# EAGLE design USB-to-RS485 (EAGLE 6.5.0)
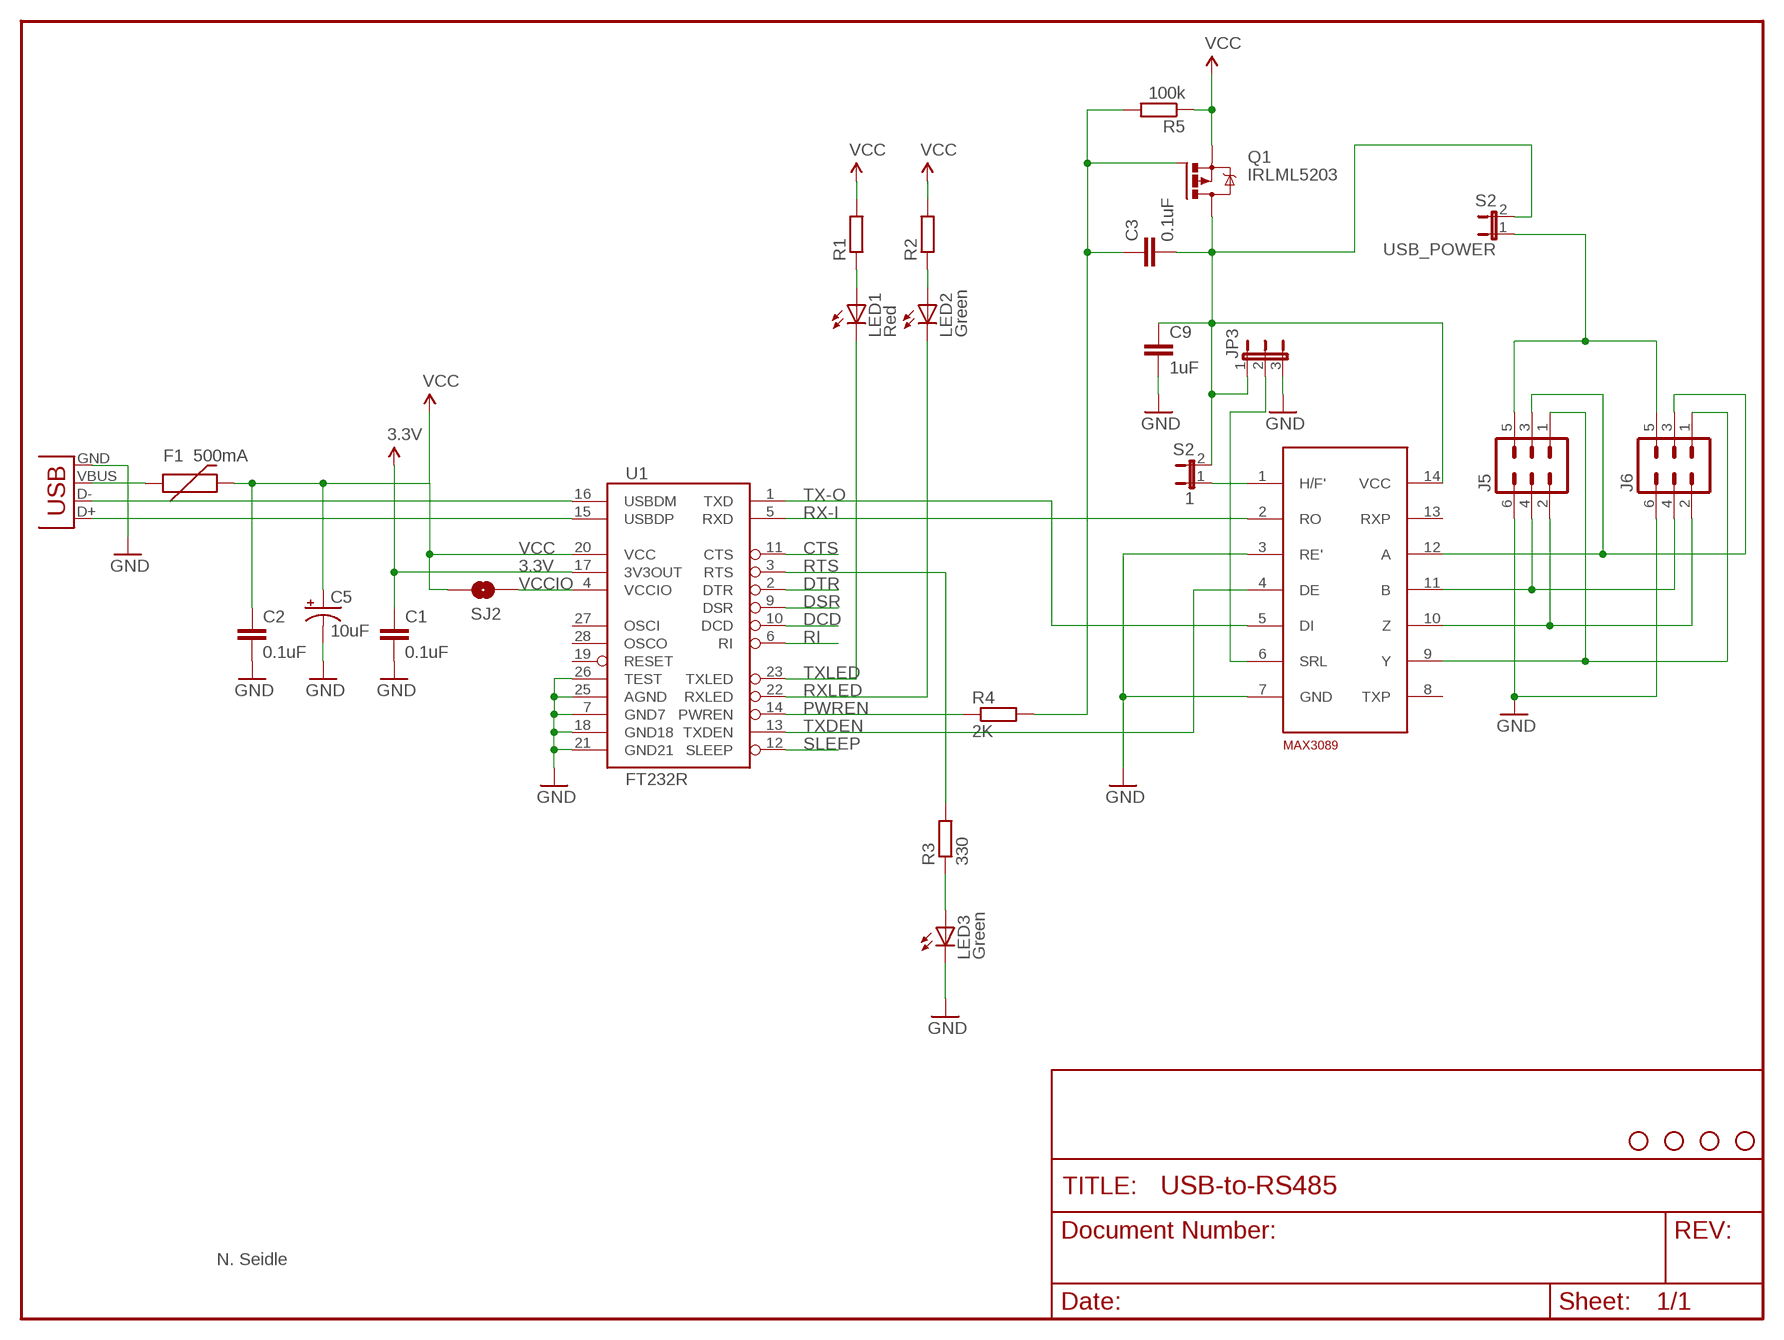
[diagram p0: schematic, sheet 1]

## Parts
1  S2  JP1E  [JP1]
C1  0.1uF  RCL_C-EUC0603  [RCL_C0603]
C2  0.1uF  RCL_C-EUC0603  [RCL_C0603]
C3  0.1uF  RCL_C-EUC0603  [RCL_C0603]
C5  10uF  CAP_POL1206  [EIA3216]
C9  1uF  RCL_C-EUC0603  [RCL_C0603]
F1  500mA  PTCSMD  [PTC-1206]
J5  ML6  [ML6]
J6  ML6  [ML6]
JP1  STAND-OFF  [STAND-OFF]
JP3  JP2E  [JP2]
JP6  STAND-OFF  [STAND-OFF]
JP7  STAND-OFF  [STAND-OFF]
JP8  STAND-OFF  [STAND-OFF]
LED1  Red  LED0603  [LED-0603]
LED2  Green  LED0603  [LED-0603]
LED3  Green  LED0603  [LED-0603]
Q1  IRLML5203  [MICRO3]
R1  RCL_R-EU_R0603  [RCL_R0603]
R2  RCL_R-EU_R0603  [RCL_R0603]
R3  330  RCL_R-EU_R0603  [RCL_R0603]
R4  2K  RCL_R-EU_R0603  [RCL_R0603]
R5  100k  RCL_R-EU_R0603  [RCL_R0603]
SJ2  SOLDERJUMPERNC2  [SJ_2S-NOTRACE]
U1  FT232R  FT232RLSSOP  [SSOP28DB]
U$4  MAX3089  [SO14]
USB_POWER  S2  JP1E  [JP1]
X2  USBSMD  [USB-MINIB]

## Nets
3.3V [power]: C1.1 U1.17(3V3OUT)
CTS: U1.11(CTS)
DCD: U1.10(DCD)
DSR: U1.9(DSR)
DTR: U1.2(DTR)
GND [power]: C1.2 C2.2 C5.C(-) C9.2 J5.6 J6.6 JP3.3 LED3.C U1.7(GND7) U1.18(GND18) U1.21(GND21) U1.25(AGND) U1.26(TEST) U$4.3(RE') U$4.7(GND) X2.GND
J5 [power]: J5.1 J6.1 U$4.9(Y)
N$1: LED1.A R1.1
N$2: LED2.A R2.1
N$3: F1.1 X2.VBUS
N$4: LED3.A R3.1
N$5 [power]: 1.2 C3.2 C9.1 JP3.1 Q1.3(D) U$4.14(VCC) USB_POWER.2
N$6 [supply]: J5.5 J6.5 USB_POWER.1
N$7: C3.1 Q1.1(G) R4.2 R5.2
N$9: JP3.2 U$4.6(SRL)
N$38 [supply]: 1.1 U$4.1(H/F')
N$41 [power]: J5.2 J6.2 U$4.10(Z)
N$48 [power]: J5.3 J6.3 U$4.12(A)
N$49 [power]: J5.4 J6.4 U$4.11(B)
PWREN: R4.1 U1.14(PWREN)
RI: U1.6(RI)
RTS: R3.2 U1.3(RTS)
RX-I: U1.5(RXD) U$4.2(RO)
RXLED: LED2.C U1.22(RXLED)
SLEEP: U1.12(SLEEP)
TX-O: U1.1(TXD) U$4.5(DI)
TXDEN: U1.13(TXDEN) U$4.4(DE)
TXLED: LED1.C U1.23(TXLED)
USB_D+: U1.15(USBDP) X2.D+
USB_D-: U1.16(USBDM) X2.D-
VCC [power]: C2.1 C5.A(+) F1.2 Q1.2(S) R1.2 R2.2 R5.1 SJ2.2 U1.20(VCC)
VCCIO: SJ2.1 U1.4(VCCIO)
Unconnected: U1.19(RESET) U1.27(OSCI) U1.28(OSCO) U$4.8(TXP) U$4.13(RXP)

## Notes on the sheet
- N. Seidle

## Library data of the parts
1 USB_POWER = jumper:JP1E: JUMPER
C1-C3 C9 = mc_rip2_1:RCL_C-EU: CAPACITOR, European symbol
C5 = SparkFun:CAP_POL: Capacitor Polarized
F1 = SparkFun:PTC: Resettable Fuse PTC
J5 J6 = con-harting-ml:ML6: HARTING
JP1 JP6-JP8 = SparkFun:STAND-OFF: Stand Off
JP3 = jumper:JP2E: JUMPER
LED1-LED3 = SparkFun:LED: LEDs
Q1 = transistor-power:IRLML5203: HEXFET P-Channel Power MOSFET
R1-R5 = mc_rip2_1:RCL_R-EU_: RESISTOR, European symbol
SJ2 = SparkFun:SOLDERJUMPER: Solder Jumper
U1 = SparkFun:FT232RL: USB UART FT232RL 4th Generation USB UART (USB <-> Serial) Controller. Spark Fun Electronics SKU : COM-00650
U$4 = maxim:MAX3089: RS485 driver
X2 = SparkFun:USB: USB Connectors USB-B-PTH is fully proven SKU : PRT-00139 USB-miniB is fully proven SKU : PRT-00587 USB-A-PCB is untested. USB-A-H is throughly reviewed, but untested. Spark Fun Electronics SKU : PRT-00437 USB-B-SMT is throughly reviewed, but untested. Needs silkscreen touching up. USB-A-S has not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

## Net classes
0 default: width 0.203 mm
1 power: width 0.254 mm
2 supply: width 0.5 mm, clearance 0.2 mm

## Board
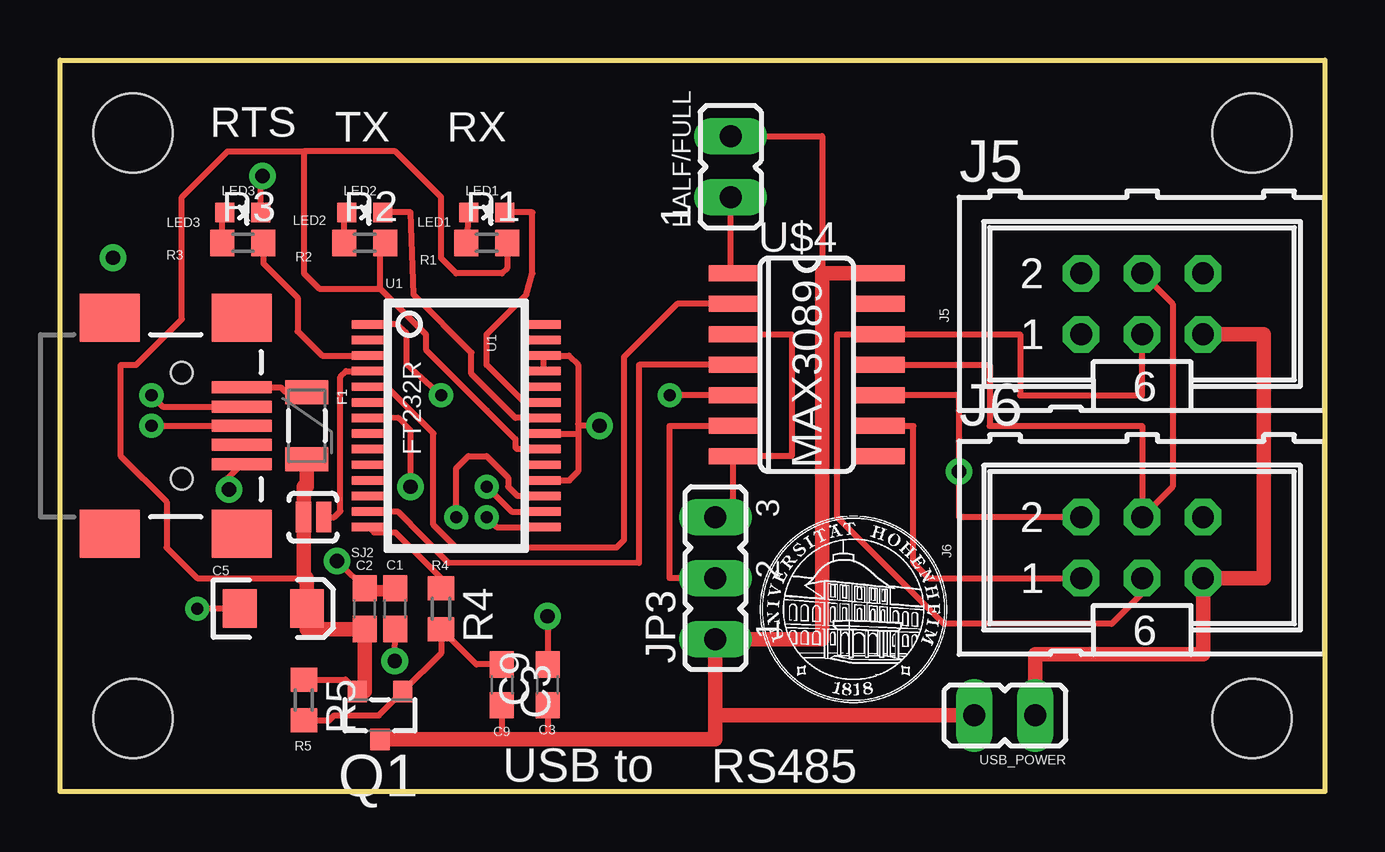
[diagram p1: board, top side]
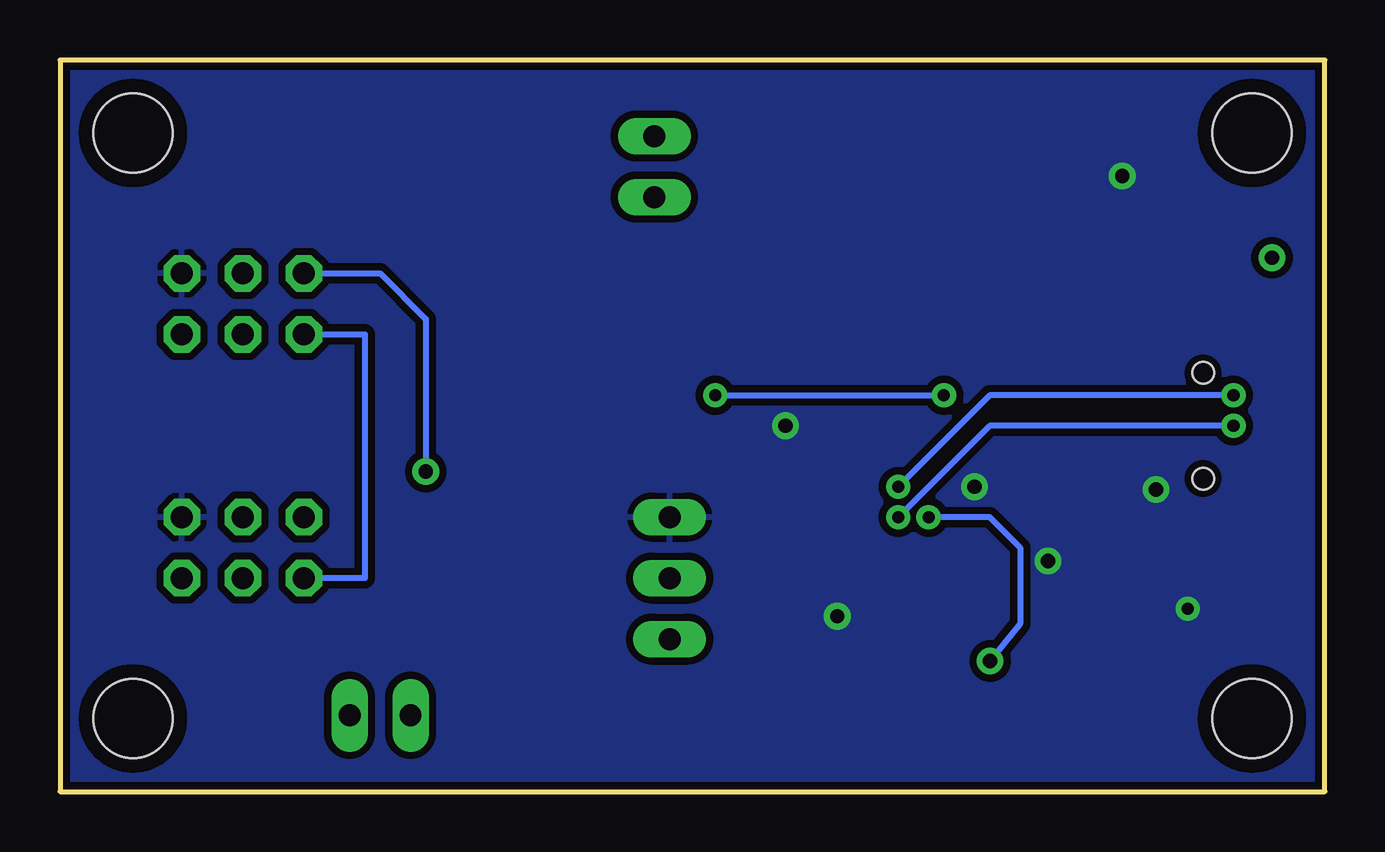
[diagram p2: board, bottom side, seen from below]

Size 52.7 x 30.48 mm. Coordinates in mm from the lower left corner, seen from the top.
Outline: 52.7,0 0,0 0,30.48 52.7,30.48 52.7,0
Copper layers (1*16): Top 0.035mm / dielectric 1.5mm / Bottom 0.035mm
Design rules "SparkFun": minimum track width 8mil, minimum drill 20mil, track to track 8mil, track to pad 8mil, pad to pad 8mil, via to via 8mil, smd to smd 8mil, copper to edge 8mil, drill to drill 8mil, minimum pad ring 12mil, minimum via ring 10mil, stop-mask expansion 4mil, vias tented up to drill 20mil, thermal gap 10mil

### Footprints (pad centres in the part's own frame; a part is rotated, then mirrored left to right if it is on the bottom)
JP1 = drill 0.914 long: 1 0,-1.27; 2 0,1.27
RCL_C0603 = smd 1.1 x 1: 1 -0.85,0; 2 0.85,0
EIA3216 = smd 1.4 x 1.6: A 1.4,0; C -1.4,0
PTC-1206 = smd 1 x 1.8: 1 -1.4,0; 2 1.4,0
ML6 = drill 0.914 octagon: 1 -2.54,-1.27; 2 -2.54,1.27; 3 0,-1.27; 4 0,1.27; 5 2.54,-1.27; 6 2.54,1.27
STAND-OFF = hole 3.302: 0,0
JP2 = drill 0.914 long: 1 -2.54,0; 2 0,0; 3 2.54,0
LED-0603 = smd 0.8 x 0.8: A 0,-0.75; C 0,0.75
MICRO3 = smd 0.8 x 0.9: 1 -0.95,-1; 2 0.95,-1; 3 0,1
RCL_R0603 = smd 1 x 1.1: 1 -0.85,0; 2 0.85,0
SJ_2S-NOTRACE = smd 0.635 x 1.27: 1 -0.45,0; 2 0.4,0
SSOP28DB = smd 0.348 x 1.397: 1 -4.225,-3.656; 2 -3.575,-3.656; 3 -2.925,-3.656; 4 -2.275,-3.656; 5 -1.625,-3.656; 6 -0.975,-3.656; 7 -0.325,-3.656; 8 0.325,-3.656; 9 0.975,-3.656; 10 1.625,-3.656; 11 2.275,-3.656; 12 2.925,-3.656; 13 3.575,-3.656; 14 4.225,-3.656; 15 4.225,3.656; 16 3.575,3.656; 17 2.925,3.656; 18 2.275,3.656; 19 1.625,3.656; 20 0.975,3.656; 21 0.325,3.656; 22 -0.325,3.656; 23 -0.975,3.656; 24 -1.625,3.656; 25 -2.275,3.656; 26 -2.925,3.656; 27 -3.575,3.656; 28 -4.225,3.656
SO14 = smd 0.66 x 2.032: 1 -3.81,-3.073; 2 -2.54,-3.073; 3 -1.27,-3.073; 4 0,-3.073; 5 1.27,-3.073; 6 2.54,-3.073; 7 3.81,-3.073; 8 3.81,3.073; 9 2.54,3.073; 10 1.27,3.073; 11 0,3.073; 12 -1.27,3.073; 13 -2.54,3.073; 14 -3.81,3.073
USB-MINIB = smd 2.5 x 0.5: D+ 2.5,0; D- 2.5,0.8; GND 2.5,-1.6; ID 2.5,-0.8; VBUS 2.5,1.6 | smd 2.5 x 2: GND@1 -3,-4.5; GND@2 -3,4.5; GND@3 2.5,4.5; GND@4 2.5,-4.5 | hole 0.9: 0,2.2; 0,-2.2

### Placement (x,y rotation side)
1  27.94,26.04 0 top
C1  13.97,7.62 90 top
C2  12.7,7.62 90 top
C3  18.41,4.45 270 top
C5  8.89,7.62 0 top
C9  20.32,4.45 90 top
F1  10.29,15.24 270 top
J5  45.09,20.32 0 top
J6  45.09,10.16 0 top
JP1  3.04,27.44 0 top
JP3  27.3,8.89 90 top
JP6  3.04,3.04 0 top
JP7  49.66,27.44 0 top
JP8  49.66,3.04 0 top
LED1  17.78,24.13 270 top
LED2  12.7,24.13 270 top
LED3  7.62,24.13 270 top
Q1  13.34,3.17 180 top
R1  17.78,22.86 0 top
R2  12.7,22.86 0 top
R3  7.62,22.86 0 top
R4  15.88,7.62 270 top
R5  10.16,3.81 270 top
SJ2  10.54,11.43 180 top
U1  16.51,15.24 270 top
U$4  31.11,17.78 270 top
USB_POWER  39.37,3.17 90 top
X2  5.08,15.24 0 top

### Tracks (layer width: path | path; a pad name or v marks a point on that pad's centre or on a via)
3.3V  (via drill 0.51, 0.6)
  Top 0.254: v16.51,11.43 16.51,13.46 17.02,13.97 17.78,13.97 18.67,13.08 18.67,12.7 19.05,12.31 U1.17 | v13.95,5.44 C1.1
  Bottom 0.254: v16.51,11.43 13.97,11.43 12.7,10.16 12.7,6.99 v13.95,5.44
GND  (via drill 0.5, 0.6)
  Top 0.254: C5.C v5.71,7.62 | U1.18 21.22,12.96 21.59,13.34 21.59,14.9 | U1.21 21.58,14.91 21.59,14.9 | 21.59,15.3 21.59,17.78 21.2,18.16 U1.26 U1.25 | 21.59,15.3 21.59,14.9 | U$4.3 30.48,19.05 30.48,13.97 U$4.7 28.04,12.17 JP3.3 | v22.48,15.24 21.65,15.24 21.59,15.3 | LED3.C 8.37,25.48 8.35,25.5 | v7.03,12.58 6.99,13.04 X2.GND | v14.61,12.7 14.61,15.03 14.09,15.57 12.86,15.56 U1.7 | 12.7,8.57 12.8,8.47 C1.2 13.76,8.26 12.7,8.26 C2.2 12.38,8.79 v11.54,9.6 | v20.32,7.3 C9.2
  Top 0.406: 8.37,25.48 8.45,25.48 v8.45,25.65
  pour Bottom (isolate 0.305): 0,30.48 52.7,30.48 52.7,0 0,0
J5
  Top 0.254: U$4.9 35.56,15.24 35.56,9.53 36.2,8.89 J6.1
  Bottom 0.254: J5.1 40.01,19.05 40.01,8.89 J6.1
N$1
  Top 0.254: LED1.A R1.1
N$2
  Top 0.254: R2.1 11.85,24.03 LED2.A
N$3
  Top 0.254: X2.VBUS 9.2,16.84 9.4,16.64 10.54,16.64 F1.1
N$4
  Top 0.254: R3.1 6.77,24.03 LED3.A
N$5
  Top 0.254: 1.2 31.75,27.3 31.75,21.59 | C3.2 18.41,2.17 | C9.1 20.32,2.17
  Top 0.61: 27.3,3.17 27.3,2.17 20.32,2.17 18.41,2.17 Q1.3 | 27.3,3.17 JP3.1 31.75,6.35 31.75,21.59 U$4.14 | USB_POWER.2 27.3,3.17
N$6
  Top 0.61: USB_POWER.1 40.64,5.71 47.62,5.71 J6.5 50.16,8.89 50.16,19.05 J5.5
N$7
  Top 0.254: C3.1 17.35,5.29 R4.2 15.88,5.76 Q1.1 13.29,3.17 11.43,3.17 11.21,2.96 R5.2
N$8  (via drill 0.6)
  other vias: 2.21,22.24
N$9
  Top 0.254: 28.57,15.24 U$4.6 25.4,15.24 25.4,8.89 JP3.2
N$38
  Top 0.254: U$4.1 27.94,21.59 1.1
N$41  (via drill 0.6)
  Top 0.254: J6.2 37.47,11.43 v37.47,13.34 37.47,16.51 U$4.10
  Bottom 0.254: J5.2 39.37,21.59 37.47,19.68 v37.47,13.34
N$48
  Top 0.254: J5.3 45.09,16.51 40.01,16.51 40.01,19.05 U$4.12 32.38,19.05 32.38,11.43 36.83,6.99 43.81,6.99 45.09,8.26 J6.3
N$49
  Top 0.254: U$4.11 38.73,17.78 38.73,15.24 45.09,15.24 J6.4 46.35,12.7 46.35,20.32 J5.4
PWREN
  Top 0.254: U1.14 13.07,10.79 13.97,10.79 15.88,8.89 R4.1
RTS
  Top 0.254: U1.3 10.92,18.16 9.91,19.18 9.91,20.57 8.47,22.01 R3.2
RX-I
  Top 0.254: U1.5 13.62,16.86 15.56,14.92 15.56,11.11 16.51,10.16 23.18,10.16 23.5,10.48 23.5,18.1 25.72,20.32 U$4.2
RXLED
  Top 0.254: U1.22 18.98,15.56 17.14,17.4 17.14,18.29 14.73,20.7 14.61,24.13 LED2.C
TX-O  (via drill 0.5)
  Top 0.254: U$4.5 v25.4,16.51 | v15.88,16.51 14.45,17.8 14.45,19.09 14.02,19.46 U1.1
  Bottom 0.254: v25.4,16.51 v15.88,16.51
TXDEN
  Top 0.254: U$4.4 24.13,17.78 24.13,9.53 16.19,9.51 14.1,11.65 U1.13
TXLED
  Top 0.254: U1.23 19.34,16.21 17.78,17.78 17.78,19.05 19.43,20.7 19.68,21.59 19.68,24.13 LED1.C
USB_D+  (via drill 0.51)
  Top 0.254: v3.81,15.24 X2.D+ | U1.15 18.2,11.02 v17.78,11.43
  Bottom 0.254: v3.81,15.24 13.97,15.24 v17.78,11.43
USB_D-  (via drill 0.51)
  Top 0.254: U1.16 18.82,11.66 v17.78,12.7 | X2.D- 4.28,16.04 v3.81,16.51
  Bottom 0.254: v17.78,12.7 13.97,16.51 v3.81,16.51
VCC
  Top 0.254: R5.1 11.9,4.66 Q1.2 | 13.34,22.86 R2.2 13.34,22.64 13.34,20.95 | 18.64,22.95 18.63,22.95 R1.2 18.63,21.8 18.41,21.59 16.51,21.59 15.88,22.23 15.88,24.77 13.97,26.67 10.16,26.67 | 10.41,13.94 10.32,13.84 F1.2 10.29,13.46 10.16,13.34 | 10.16,13.34 10.16,13.97 | 10.16,13.34 10.16,12.7 | 10.16,26.67 6.99,26.67 5.08,24.77 5.08,19.68 3.17,17.78 2.54,17.78 2.54,13.97 4.45,12.06 4.45,10.16 5.71,8.89 10.16,8.89 | 10.16,26.67 10.16,21.59 10.79,20.95 13.34,20.95 | 13.34,20.95 15.24,19.05 15.24,18.41 17.78,15.88 17.79,15.88 18.98,14.69 18.98,14.34 19.04,14.27 20.16,14.27 U1.20
  Top 0.61: 10.16,11.43 10.16,12.7 10.29,12.7 F1.2 | SJ2.2 10.16,11.43 | 10.16,11.43 10.16,8.89 10.29,8.89 C5.A 10.29,6.77 C2.1 12.7,4.17 Q1.2
VCCIO
  Top 0.254: SJ2.1 11.43,11.43 11.68,11.68 11.68,17.27 11.93,17.52 U1.4

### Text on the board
t_silke: RTS | TX | RX | LED3 | LED2 | LED1 | R3 | HALF/FULL | R2 | R1 | U1 | MAX3089 | 2 | J5 | FT232R | 1 | F1 | 6 | 2 | SJ2 | J6 | C5 | C2 | C1 | R4 | 1 | 6 | C9 | R5 | C3 | USB_POWER | USB to | RS485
